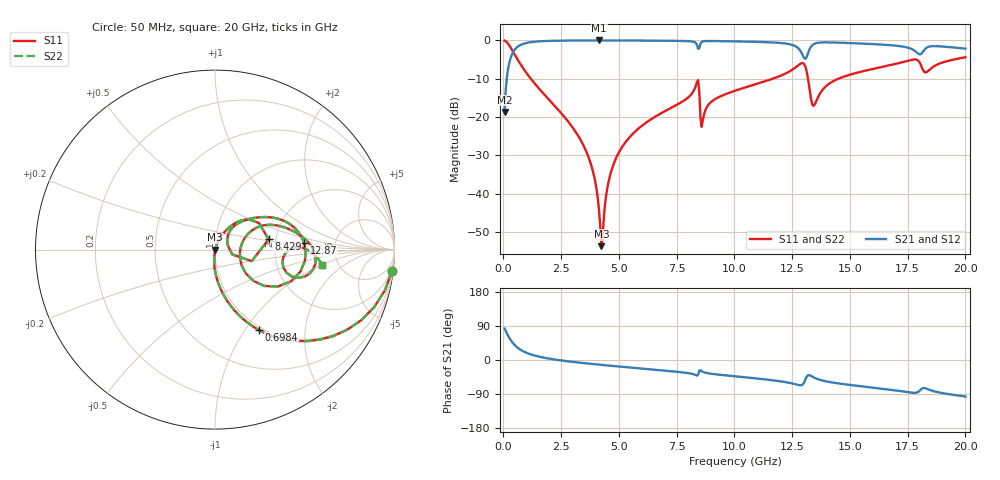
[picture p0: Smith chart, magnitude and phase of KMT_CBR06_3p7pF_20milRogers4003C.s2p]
! Data measured by Modelithics Inc. support@modelithics.com 813-866-6335
! KEMET CBR0603 3.7pF, Pad Width= 0.851mm, Pad Length= 0.64mm, Pad Gap= 0.62mm, 20mil Rogers 4003C substrate Data, January 2022
# hz S ma R 50
! 2 Port Network Data from SP1.SP block
! freq  magS11  angS11  magS21  angS21  magS12  angS12  magS22  angS22
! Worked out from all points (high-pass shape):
!   401 points, 50 MHz to 20 GHz, reference 50 ohm
!   highest |S21| = -0.02 dB at 4.14 GHz (marker M1); lowest = -18.7 dB at 50 MHz (marker M2)
!   |S21| within 3 dB of the highest: 423.9 MHz to 12.88 GHz (12.46 GHz wide, 187 % of centre); 13.2 GHz to 17.87 GHz (4.667 GHz wide, 30 % of centre)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
!   lowest |S11| = -53.7 dB at 4.239 GHz (marker M3), VSWR 1.00, Z = 50.2 - j0.115 ohm
!   |S11| at or under -10 dB: 1.184 GHz to 11.65 GHz (10.47 GHz wide, 163 % of centre); 13.18 GHz to 14.5 GHz (1.318 GHz wide, 9.52 % of centre)
!   |S22| runs from -53.7 to -0.1 dB; largest |S21 - S12| = 0
!   S11 on the Smith chart (normalised r, x): 50 MHz: 1, -17; 698.4 MHz: 0.96, -1.16; 8.429 GHz: 1.83, +0.23; 12.87 GHz: 2.95, +0.29; 20 GHz: 3.77, -0.99
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5e7  0.9932 -6.8  0.1164 83.2  0.1164 83.2  0.9932 -6.8
2.99375e8  0.817 -36.1  0.5759 53.9  0.5759 53.9  0.817 -36.1
6.98375e8  0.5111 -61.3  0.8586 28.6  0.8586 28.6  0.5111 -61.3
1.496375e9  0.2434 -80.2  0.9687 9.5  0.9687 9.5  0.2434 -80.2
3.391625e9  0.0471 -95.5  0.997 -7.6  0.997 -7.6  0.0471 -95.5
3.890375e9  0.01872 -95.1  0.9978 -10.8  0.9978 -10.8  0.01872 -95.1
4.13975e9  0.006026 -83.7  0.9979 -12.3  0.9979 -12.3  0.006026 -83.7
4.2395e9  0.002074 -33.6  0.9979 -12.9  0.9979 -12.9  0.002074 -33.6
4.588625e9  0.01613 67.9  0.9977 -14.9  0.9977 -14.9  0.01613 67.9
4.93775e9  0.03194 69.4  0.9972 -16.9  0.9972 -16.9  0.03194 69.4
6.73325e9  0.1083 61.9  0.9912 -26.7  0.9912 -26.7  0.1083 61.9
8.429e9  0.3041 10.9  0.7761 -39.0  0.7761 -39.0  0.3041 10.9
8.6285e9  0.09033 40.9  0.968 -31.0  0.968 -31.0  0.09033 40.9
1.0025e10  0.2206 45.9  0.9708 -43.0  0.9708 -43.0  0.2206 45.9
1.286788e10  0.4981 4.3  0.7198 -66.8  0.7198 -66.8  0.4981 4.3
1.311725e10  0.407 -30.3  0.601 -45.5  0.601 -45.5  0.407 -30.3
1.336662e10  0.1475 -19.0  0.8635 -43.6  0.8635 -43.6  0.1475 -19.0
1.416462e10  0.2805 27.4  0.9403 -58.7  0.9403 -58.7  0.2805 27.4
1.670825e10  0.4732 10.4  0.8677 -78.0  0.8677 -78.0  0.4732 10.4
1.805488e10  0.4914 -18.7  0.6598 -78.9  0.6598 -78.9  0.4914 -18.7
1.86035e10  0.4518 1.6  0.8421 -81.9  0.8421 -81.9  0.4518 1.6
2e10  0.6038 -7.9  0.7802 -96.4  0.7802 -96.4  0.6038 -7.9
